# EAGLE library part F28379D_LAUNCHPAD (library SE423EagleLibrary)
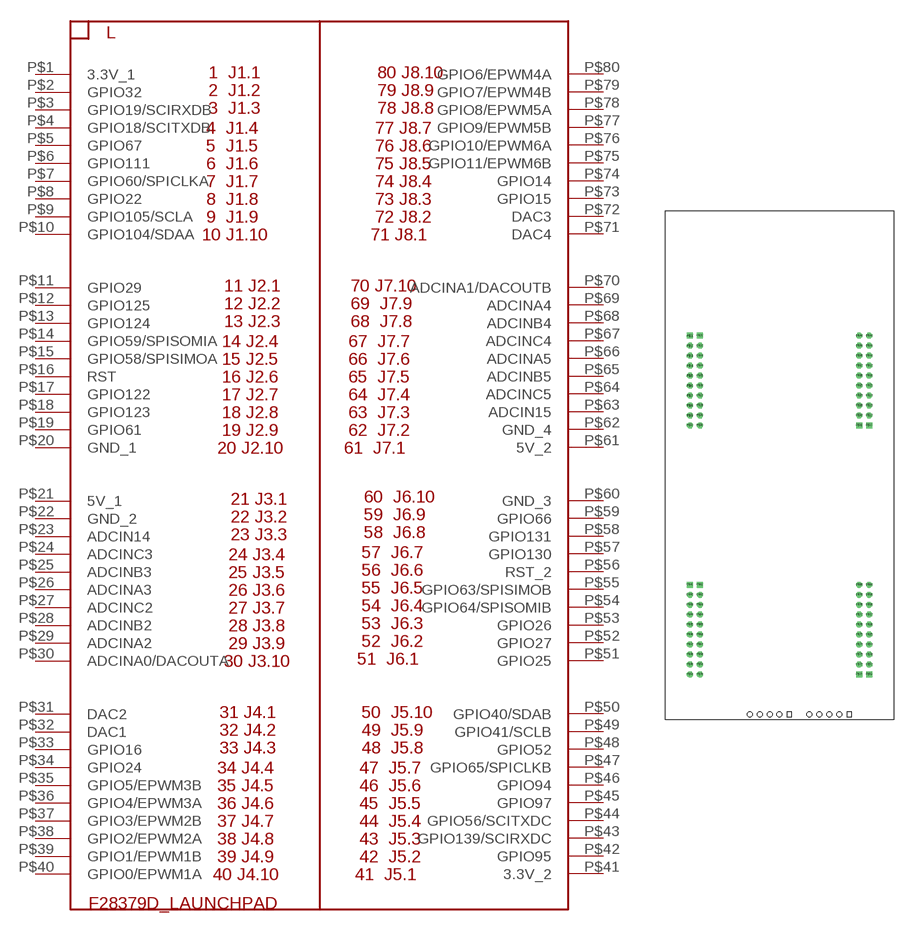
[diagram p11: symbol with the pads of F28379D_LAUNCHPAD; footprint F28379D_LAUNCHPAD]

Designator prefix L

## F28379D_LAUNCHPAD  [F28379D_LAUNCHPAD]
P$1  3.3V_1
P$2  GPIO32
P$3  GPIO19/SCIRXDB
P$4  GPIO18/SCITXDB
P$5  GPIO67
P$6  GPIO111
P$7  GPIO60/SPICLKA
P$8  GPIO22
P$9  GPIO105/SCLA
P$10  GPIO104/SDAA
P$11  GPIO29
P$12  GPIO125
P$13  GPIO124
P$14  GPIO59/SPISOMIA
P$15  GPIO58/SPISIMOA
P$16  RST
P$17  GPIO122
P$18  GPIO123
P$19  GPIO61
P$20  GND_1
P$21  5V_1
P$22  GND_2
P$23  ADCIN14
P$24  ADCINC3
P$25  ADCINB3
P$26  ADCINA3
P$27  ADCINC2
P$28  ADCINB2
P$29  ADCINA2
P$30  ADCINA0/DACOUTA
P$31  DAC2
P$32  DAC1
P$33  GPIO16
P$34  GPIO24
P$35  GPIO5/EPWM3B
P$36  GPIO4/EPWM3A
P$37  GPIO3/EPWM2B
P$38  GPIO2/EPWM2A
P$39  GPIO1/EPWM1B
P$40  GPIO0/EPWM1A
P$41  3.3V_2
P$42  GPIO95
P$43  GPIO139/SCIRXDC
P$44  GPIO56/SCITXDC
P$45  GPIO97
P$46  GPIO94
P$47  GPIO65/SPICLKB
P$48  GPIO52
P$49  GPIO41/SCLB
P$50  GPIO40/SDAB
P$51  GPIO25
P$52  GPIO27
P$53  GPIO26
P$54  GPIO64/SPISOMIB
P$55  GPIO63/SPISIMOB
P$56  RST_2
P$57  GPIO130
P$58  GPIO131
P$59  GPIO66
P$60  GND_3
P$61  5V_2
P$62  GND_4
P$63  ADCIN15
P$64  ADCINC5
P$65  ADCINB5
P$66  ADCINA5
P$67  ADCINC4
P$68  ADCINB4
P$69  ADCINA4
P$70  ADCINA1/DACOUTB
P$71  DAC4
P$72  DAC3
P$73  GPIO15
P$74  GPIO14
P$75  GPIO11/EPWM6B
P$76  GPIO10/EPWM6A
P$77  GPIO9/EPWM5B
P$78  GPIO8/EPWM5A
P$79  GPIO7/EPWM4B
P$80  GPIO6/EPWM4A

## Footprint F28379D_LAUNCHPAD (pad centres in mm)
drill 1.016 square: P$1 -24.13,33.02; P$11 21.59,10.16; P$21 -21.59,33.02; P$31 19.05,10.16; P$41 -24.13,-30.48; P$51 21.59,-53.34; P$61 -21.59,-30.48; P$71 19.05,-53.34
drill 1.016 octagon: P$2 -24.13,30.48; P$3 -24.13,27.94; P$4 -24.13,25.4; P$5 -24.13,22.86; P$6 -24.13,20.32; P$7 -24.13,17.78; P$8 -24.13,15.24; P$9 -24.13,12.7; P$10 -24.13,10.16; P$12 21.59,12.7; P$13 21.59,15.24; P$14 21.59,17.78; P$15 21.59,20.32; P$16 21.59,22.86; P$17 21.59,25.4; P$18 21.59,27.94; P$19 21.59,30.48; P$20 21.59,33.02; P$22 -21.59,30.48; P$23 -21.59,27.94; P$24 -21.59,25.4; P$25 -21.59,22.86; P$26 -21.59,20.32; P$27 -21.59,17.78; P$28 -21.59,15.24; P$29 -21.59,12.7; P$30 -21.59,10.16; P$32 19.05,12.7; P$33 19.05,15.24; P$34 19.05,17.78; P$35 19.05,20.32; P$36 19.05,22.86; P$37 19.05,25.4; P$38 19.05,27.94; P$39 19.05,30.48; P$40 19.05,33.02; P$42 -24.13,-33.02; P$43 -24.13,-35.56; P$44 -24.13,-38.1; P$45 -24.13,-40.64; P$46 -24.13,-43.18; P$47 -24.13,-45.72; P$48 -24.13,-48.26; P$49 -24.13,-50.8; P$50 -24.13,-53.34; P$52 21.59,-50.8; P$53 21.59,-48.26; P$54 21.59,-45.72; P$55 21.59,-43.18; P$56 21.59,-40.64; P$57 21.59,-38.1; P$58 21.59,-35.56; P$59 21.59,-33.02; P$60 21.59,-30.48; P$62 -21.59,-33.02; P$63 -21.59,-35.56; P$64 -21.59,-38.1; P$65 -21.59,-40.64; P$66 -21.59,-43.18; P$67 -21.59,-45.72; P$68 -21.59,-48.26; P$69 -21.59,-50.8; P$70 -21.59,-53.34; P$72 19.05,-50.8; P$73 19.05,-48.26; P$74 19.05,-45.72; P$75 19.05,-43.18; P$76 19.05,-40.64; P$77 19.05,-38.1; P$78 19.05,-35.56; P$79 19.05,-33.02; P$80 19.05,-30.48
